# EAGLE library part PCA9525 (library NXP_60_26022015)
The PCA9525 is a monolithic CMOS integrated circuit for bus buffering in applications including I2C-bus, SMBus, DDC, PMBus, and other systems based on similar principles. AAL Eindhoven MK
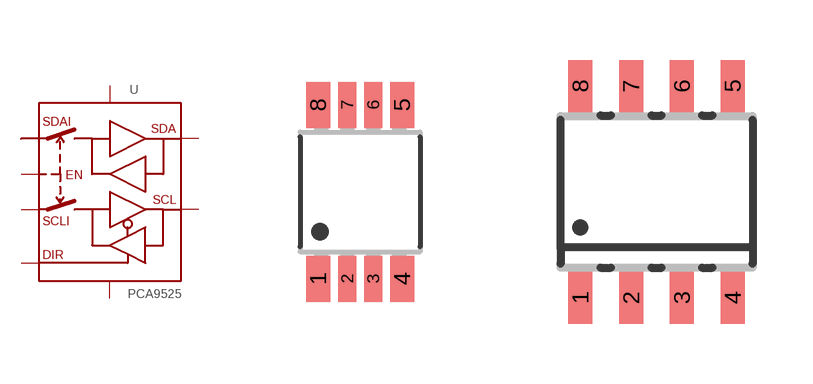
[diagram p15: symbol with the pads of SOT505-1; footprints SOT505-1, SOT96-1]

Designator prefix U

## PCA9525DP  [SOT505-1]
1  EN  in
2  SCL
3  SCLI
4  VDD  pwr
5  DIR  in
6  SDAI
7  SDA
8  VSS  pwr

## PCA9525P  [SOT96-1]
Pads as for SOT505-1

## Footprint SOT505-1 (pad centres in mm)
SOT505-1 TSSOP8: plastic thin shrink small outline package; 8 leads; body width 3 mm JEDEC: -- IEC: --
smd 0.6 x 1.15: 1 -1.05,-2.175; 4 1.05,-2.175; 5 1.05,2.175; 8 -1.05,2.175
smd 0.45 x 1.15: 2 -0.325,-2.175; 3 0.325,-2.175; 6 0.325,2.175; 7 -0.325,2.175

## Footprint SOT96-1 (pad centres in mm)
SOT96-1 SO8: plastic small outline package; 8 leads; body width 3.9 mm JEDEC: MS-012 IEC: 076E03
smd 0.6 x 1.3: 1 -1.905,-2.65; 2 -0.635,-2.65; 3 0.635,-2.65; 4 1.905,-2.65; 5 1.905,2.65; 6 0.635,2.65; 7 -0.635,2.65; 8 -1.905,2.65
